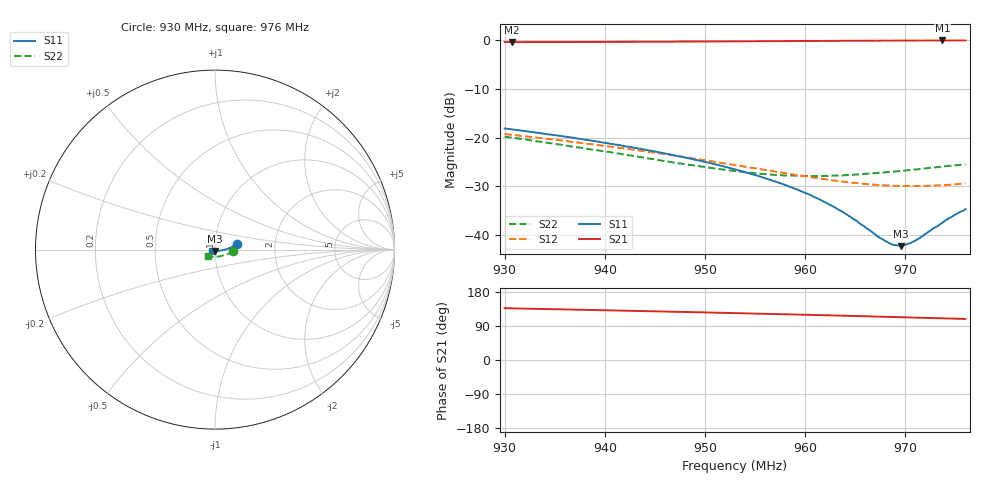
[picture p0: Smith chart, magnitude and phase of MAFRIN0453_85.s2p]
!Part Number:  MAFRIN0453
!Name:  MariaCraven
!Comments:  1
!Thu 30/Sep/2004  1:14:14 PM
!Temperature:  85
# MHZ  S  DB  R  50
!Freq  S11(dB)  S11(ang)  S21(dB)  S21(ang)  S12(dB)  S12(ang)  S22(dB)  S22(ang)
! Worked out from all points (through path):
!   201 points, 930 MHz to 976 MHz, reference 50 ohm
!   highest |S21| = -0.07 dB at 973.7 MHz (marker M1); lowest = -0.4 dB at 930.69 MHz (marker M2)
!   group delay of S21, straight-line fit = 1.7 ns
!   lowest |S11| = -42.2 dB at 969.56 MHz (marker M3), VSWR 1.02, Z = 50 - j0.773 ohm
!   |S11| at or under -10 dB: start of sweep to end of sweep
!   |S22| runs from -27.9 to -19.8 dB; largest |S21 - S12| = 0.97
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930  -18.12 13.6  -0.40 136.8  -19.26 99.9  -19.80 -5.8
930.69  -18.30 13.0  -0.41 136.3  -19.42 99.8  -20.00 -6.6
937.82  -20.34 8.9  -0.38 132.4  -21.12 98.8  -22.13 -17.0
941.5  -21.52 6.6  -0.36 130.4  -22.08 98.9  -23.30 -23.6
945.41  -22.98 3.8  -0.33 128.2  -23.21 99.8  -24.60 -32.2
949.09  -24.52 1.0  -0.30 126.0  -24.32 101.4  -25.76 -42.4
953  -26.47 -2.8  -0.26 123.7  -25.60 104.4  -26.84 -55.0
955.3  -27.82 -5.5  -0.23 122.4  -26.36 107.0  -27.34 -63.7
957.83  -29.54 -9.2  -0.20 120.8  -27.22 110.5  -27.71 -73.8
960.82  -32.07 -15.2  -0.17 118.9  -28.17 116.2  -27.87 -86.3
962.66  -33.92 -20.6  -0.15 117.7  -28.71 120.6  -27.79 -93.8
963.81  -35.26 -25.0  -0.15 116.9  -29.00 123.3  -27.71 -98.4
965.19  -37.10 -32.2  -0.12 116.0  -29.33 127.1  -27.54 -103.7
967.26  -40.26 -50.7  -0.12 114.7  -29.68 133.0  -27.21 -111.4
968.41  -41.63 -67.2  -0.11 113.8  -29.78 136.5  -27.01 -115.5
968.87  -41.99 -74.5  -0.10 113.4  -29.86 138.1  -26.94 -116.9
969.56  -42.23 -88.3  -0.10 113.0  -29.87 140.4  -26.80 -119.2
970.48  -41.65 -106.4  -0.09 112.3  -29.89 143.2  -26.63 -122.0
971.17  -40.91 -118.3  -0.09 111.8  -29.91 145.5  -26.49 -124.1
973.7  -37.38 -148.0  -0.07 110.1  -29.75 153.4  -25.90 -131.3
975.08  -35.65 -156.1  -0.07 109.0  -29.54 157.4  -25.62 -134.7
976  -34.65 -160.5  -0.07 108.4  -29.40 159.8  -25.44 -136.8
